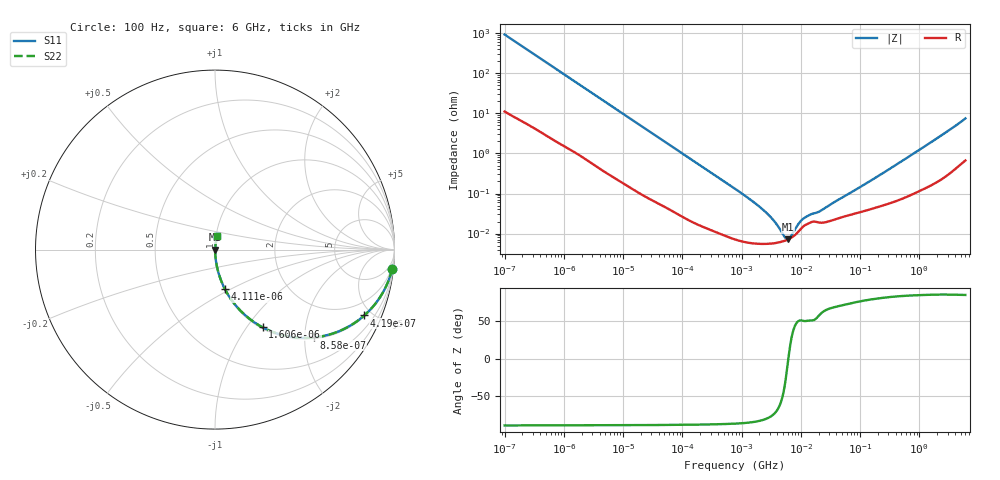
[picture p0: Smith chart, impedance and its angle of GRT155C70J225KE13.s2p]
!Murata Part Number: GRT155C70J225KE13
!These Parameters are Measured in Series Mode Connection
!Data Generated on Jun 19, 2026
!  o--ll--o
!Port1  Port2
!  o------o
!Operation Temp=25[degC], DC Bias Voltage=0[V]
!Freq. Start=100[Hz] Stop=6[GHz] 401[Steps]
# Hz S RI R 50
!Freq.(Hz) S11(Real) S11(Imag) S21(Real) S21(Imag) S12(Real) S12(Imag) S22(Real) S22(Imag)
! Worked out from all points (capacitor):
!   401 points, 100 Hz to 6 GHz, reference 50 ohm
!   read as one part in series: C = 1.7 uF near 109 Hz
!   lowest |Z| = 7.17 mohm at 6.075 MHz (marker M1)
!   series resonance near 6.167 MHz, so ESL is about 390 pH
!   S11 on the Smith chart (normalised r, x): 100 Hz: 1, -19; 419 Hz: 1.07, -4.50; 858 Hz: 1.03, -2.21; 1.606 kHz: 1.02, -1.19; 4.111 kHz: 1.01, -0.47; 6 GHz: 1.01, +0.15
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100  0.9874 -0.1058  0.0126 0.1058  0.0126 0.1058  0.9874 -0.1058
224  0.9434 -0.2245  0.0566 0.2245  0.0566 0.2245  0.9434 -0.2245
419  0.8316 -0.3669  0.1684 0.3669  0.1684 0.3669  0.8316 -0.3669
600  0.7108 -0.4459  0.2892 0.4459  0.2892 0.4459  0.7108 -0.4459
858  0.55 -0.4897  0.45 0.4897  0.45 0.4897  0.55 -0.4897
1606  0.2654 -0.4331  0.7346 0.4331  0.7346 0.4331  0.2654 -0.4331
2008  0.1898 -0.3836  0.8102 0.3836  0.8102 0.3836  0.1898 -0.3836
4111  0.0558 -0.221  0.9442 0.221  0.9442 0.221  0.0558 -0.221
11009  0.00943 -0.0877  0.9906 0.0877  0.9906 0.0877  0.00943 -0.0877
40335  0.00115 -0.0245  0.9988 0.0245  0.9988 0.0245  0.00115 -0.0245
774597  7.32e-05 -0.00132  0.9999 0.00132  0.9999 0.00132  7.32e-05 -0.00132
2481164  5.54e-05 -0.000353  0.9999 0.000353  0.9999 0.000353  5.54e-05 -0.000353
3394479  5.7e-05 -0.000215  0.9999 0.000215  0.9999 0.000215  5.7e-05 -0.000215
4856642  6.32e-05 -8.2e-05  0.9999 8.2e-05  0.9999 8.2e-05  6.32e-05 -8.2e-05
6075234  7.15e-05 -5e-06  0.9999 5e-06  0.9999 5e-06  7.15e-05 -5e-06
7266822  8.31e-05 5.63e-05  0.9999 -5.63e-05  0.9999 -5.63e-05  8.31e-05 5.63e-05
1.039699e7  0.000139 0.00017  0.9999 -0.00017  0.9999 -0.00017  0.000139 0.00017
1.555665e7  0.000197 0.000242  0.9998 -0.000242  0.9998 -0.000242  0.000197 0.000242
2.128304e7  0.000187 0.000315  0.9998 -0.000315  0.9998 -0.000315  0.000187 0.000315
3.124326e8  0.000581 0.00403  0.9994 -0.00403  0.9994 -0.00403  0.000581 0.00403
1.95892e9  0.00244 0.0233  0.9976 -0.0233  0.9976 -0.0233  0.00244 0.0233
6e9  0.0121 0.0733  0.9879 -0.0733  0.9879 -0.0733  0.0121 0.0733
